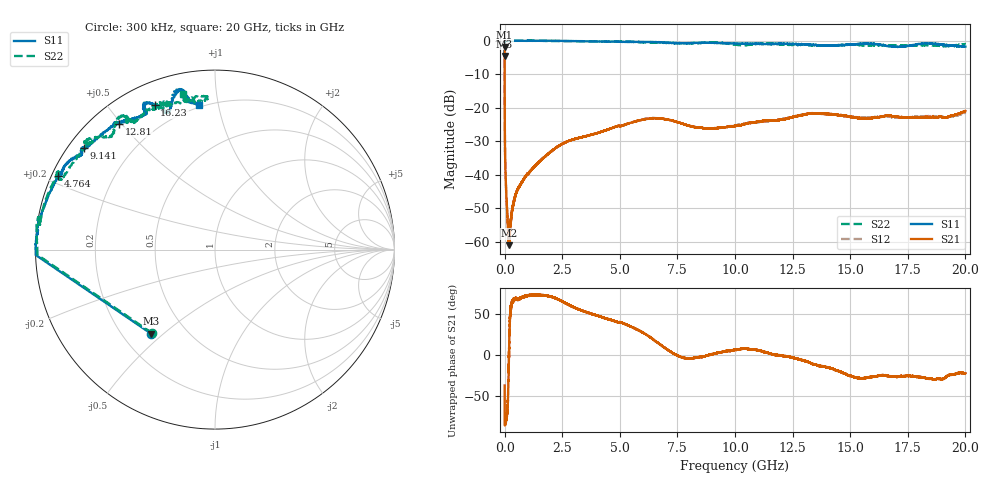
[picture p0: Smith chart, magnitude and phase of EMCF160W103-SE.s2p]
!EMCF160W103
!Johanson Technology Inc.
!www.johansontechnology.com
!Test Board Conditions:
!Substrate Type  RO4350B
!Substrate Thickness  6.6 mil
!Substrate Dk  3.66
!TL Type: GCPW
!TL Trace Width  13 mil
!TL Gap  7.5 mil
!PART MODE SINGLE ENDED (AKA BYPASS)
!DUT TOPOLOGY	SERIES-SHUNT
# MHz S  dB  R 50
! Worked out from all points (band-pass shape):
!   20001 points, 300 kHz to 20 GHz, reference 50 ohm
!   highest |S21| = -1.93 dB at 300 kHz (marker M1); lowest = -61.0 dB at 196.3 MHz (marker M2)
!   |S21| within 3 dB of the highest: start of sweep to 655.2 kHz
!   lowest |S11| = -4.6 dB at 300 kHz (marker M3), VSWR 3.86, Z = 15.9 - j22.7 ohm
!   |S11| at or under -10 dB: nowhere
!   |S22| runs from -4.7 to 0.1 dB; largest |S21 - S12| = 0.0049
!   S11 on the Smith chart (normalised r, x): 300 kHz: 0.32, -0.45; 4.764 GHz: 0.02, +0.22; 9.141 GHz: 0.04, +0.34; 12.81 GHz: 0.08, +0.49; 16.23 GHz: 0.10, +0.66; 20 GHz: 0.18, +0.88
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0.3  -4.61 -127.3  -1.93 -36.7  -1.89 -36.7  -4.70 -127.2
107.298  -0.01 179.1  -50.46 -70.2  -50.37 -69.6  -0.09 179.3
147.298  -0.01 178.5  -56.52 -52.3  -55.81 -52.8  -0.09 178.8
196.297  -0.01 178.0  -60.97 7.8  -60.02 10.1  -0.07 178.3
247.296  -0.02 177.9  -56.08 49.3  -55.76 50.8  -0.06 177.4
486.293  -0.03 176.1  -45.79 68.6  -45.62 67.7  -0.03 174.9
916.286  -0.07 173.9  -40.33 71.4  -40.38 71.1  0.04 171.6
2205.267  -0.04 171.2  -32.04 68.9  -31.98 68.6  -0.11 171.9
3334.25  -0.17 164.7  -28.80 54.3  -28.82 54.2  -0.14 163.1
4764.229  -0.29 154.8  -25.76 41.3  -25.82 41.2  -0.23 153.5
6667.2  -0.47 148.4  -23.19 14.8  -23.17 14.5  -0.62 150.9
7861.182  -0.76 144.5  -25.08 -3.6  -25.06 -3.3  -0.77 139.0
9141.163  -0.69 142.2  -26.08 2.0  -26.17 2.6  -0.55 139.8
10000.15  -0.88 138.1  -25.42 6.5  -25.25 6.7  -1.24 133.9
11465.13  -1.02 128.3  -23.77 2.5  -23.97 3.0  -0.85 125.1
12806.11  -1.11 127.3  -22.33 -5.5  -22.26 -5.4  -1.18 124.5
13334.1  -1.27 123.5  -21.69 -10.3  -21.60 -10.8  -1.39 123.1
15378.07  -1.02 116.5  -23.12 -27.5  -22.88 -27.0  -1.34 108.3
16231.06  -1.20 112.7  -22.82 -24.8  -22.81 -27.1  -1.39 110.6
16667.05  -1.67 110.4  -22.42 -25.2  -22.68 -26.5  -1.36 113.2
18602.02  -0.85 101.8  -22.75 -29.1  -22.54 -30.4  -1.43 93.1
20000  -1.80 96.2  -20.96 -22.0  -21.38 -21.3  -1.08 101.5
